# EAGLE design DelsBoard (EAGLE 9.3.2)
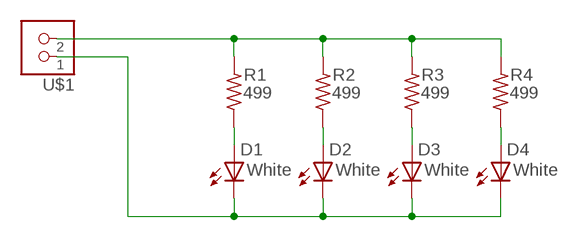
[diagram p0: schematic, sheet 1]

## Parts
D1  White  LED  [LED1206]
D2  White  LED  [LED1206]
D3  White  LED  [LED1206]
D4  White  LED  [LED1206]
R1  499  RES-US1206  [R1206]
R2  499  RES-US1206  [R1206]
R3  499  RES-US1206  [R1206]
R4  499  RES-US1206  [R1206]
U$1  HEADERPIN_X2  [1X02SMD]

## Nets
N$1: D1.1(A) R1.1
N$2: R1.2 R2.2 R3.2 R4.2 U$1.2
N$3: D2.1(A) R2.1
N$4: D3.1(A) R3.1
N$5: D4.1(A) R4.1
N$6: D1.2(C) D2.2(C) D3.2(C) D4.2(C) U$1.1

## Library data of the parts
D1-D4 = Fablab:LED: LED
R1-R4 = Fablab:RES-US: Resistor (US Symbol)
U$1 = Fablab:HEADERPIN_X2

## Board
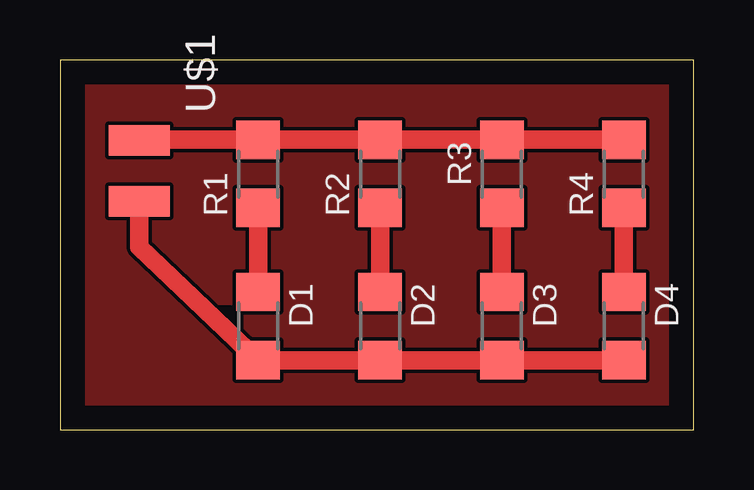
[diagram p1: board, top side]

Size 26.4 x 15.42 mm. Coordinates in mm from the lower left corner, seen from the top.
Outline: 0,0 26.4,0 26.4,15.42 0,15.42 0,0
Copper layers (1*16): Top 0.035mm / dielectric 1.5mm / Bottom 0.035mm
Design rules "default": minimum track width 6mil, minimum drill 0.35mm, track to track 6mil, track to pad 6mil, pad to pad 6mil, via to via 6mil, smd to smd 6mil, copper to edge 40mil, drill to drill 6mil, minimum pad ring 10mil, minimum via ring 8mil, stop-mask expansion 4mil, vias tented up to drill 0mil, thermal gap 10mil

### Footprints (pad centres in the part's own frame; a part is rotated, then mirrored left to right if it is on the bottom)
LED1206 = smd 1.6 x 1.803: 1 -1.422,0; 2 1.422,0
R1206 = smd 1.6 x 1.803: 1 -1.422,0; 2 1.422,0
1X02SMD = smd 2.54 x 1.27: 1 0,3.81; 2 0,1.27

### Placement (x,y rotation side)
D1  8.26,4.32 270 top
D2  13.33,4.32 270 top
D3  18.41,4.32 270 top
D4  23.49,4.32 270 top
R1  8.26,10.67 90 top
R2  13.33,10.67 90 top
R3  18.41,10.67 90 top
R4  23.49,10.67 90 top
U$1  3.3,13.33 180 top

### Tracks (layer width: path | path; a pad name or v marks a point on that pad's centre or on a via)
N$1
  Top 0.762: R1.1 D1.1
N$2
  Top 0.762: U$1.2 3.3,12.09 R1.2 R2.2 R3.2 R4.2
N$3
  Top 0.762: R2.1 D2.1
N$4
  Top 0.762: R3.1 D3.1
N$5
  Top 0.762: R4.1 D4.1
N$6
  Top 0.762: D4.2 D3.2 D2.2 D1.2 3.3,7.62 U$1.1
N$7
  pour Top: -0.13,0 26.29,0 26.29,15.37 0,15.37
